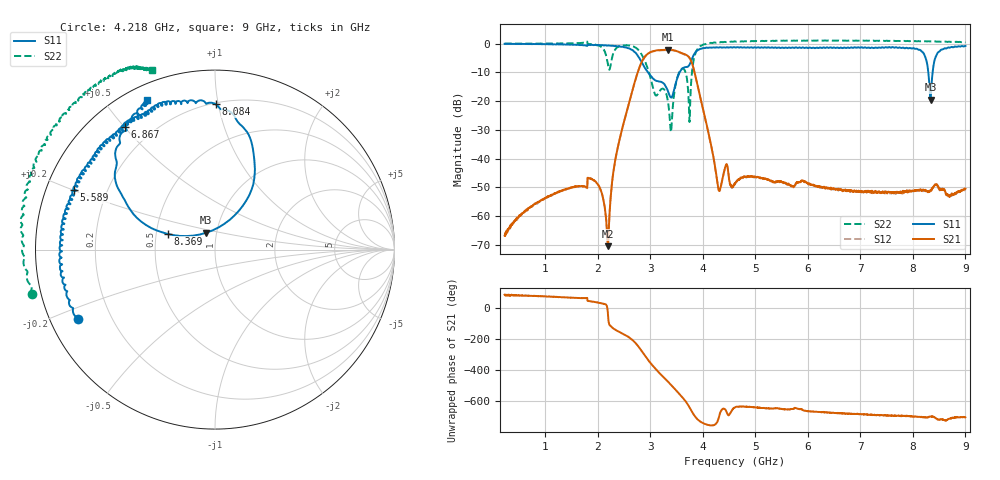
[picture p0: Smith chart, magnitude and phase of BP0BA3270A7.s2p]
!Agilent Technologies,E8358A,US41080443,A.07.50.56
!Agilent E8358A: A.07.50.56
!Date: Friday, July 21, 2017 20:19:28
!Correction: S11(Full 2 Port(1,2))
!S21(Full 2 Port(1,2))
!S12(Full 2 Port(1,2))
!S22(Full 2 Port(1,2))
!S2P File: Measurements: S11, S21, S12, S22:
# Hz S  dB  R 50
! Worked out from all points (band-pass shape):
!   1601 points, 225 MHz to 9 GHz, reference 50 ohm
!   highest |S21| = -2.10 dB at 3.329 GHz (marker M1); lowest = -70.5 dB at 2.194 GHz (marker M2)
!   |S21| within 3 dB of the highest: 2.874 GHz to 3.754 GHz (880.4 MHz wide, 26.6 % of centre)
!   lowest |S11| = -19.5 dB at 8.336 GHz (marker M3), VSWR 1.24, Z = 44.6 + j8.49 ohm
!   |S11| at or under -10 dB: 2.957 GHz to 3.557 GHz (600.2 MHz wide, 18.4 % of centre); 8.294 GHz to 8.376 GHz (81.74 MHz wide, 0.981 % of centre)
!   |S22| runs from -30.7 to 1.1 dB; largest |S21 - S12| = 0.013
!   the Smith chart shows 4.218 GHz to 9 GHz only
!   S11 on the Smith chart (normalised r, x): 4.218 GHz: 0.08, -0.24; 5.589 GHz: 0.08, +0.20; 6.867 GHz: 0.10, +0.50; 8.084 GHz: 0.21, +0.98; 8.369 GHz: 0.57, +0.11; 9 GHz: 0.06, +0.64
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2.25e8  -0.06 177.7  -66.77 84.5  -66.93 81.4  0.01 176.3
1.689328e9  -0.45 148.5  -49.57 63.0  -49.56 62.4  0.30 159.0
2.023875e9  -0.47 144.6  -49.59 32.3  -49.65 32.2  -0.69 91.9
2.193891e9  -0.64 135.6  -70.46 -48.2  -69.48 -43.5  -7.36 -8.7
2.347453e9  -0.80 122.5  -38.94 -144.4  -39.01 -144.2  -1.64 162.5
2.753297e9  -3.99 20.3  -10.29 119.6  -10.36 119.3  -1.83 73.8
2.906859e9  -8.73 -86.0  -4.28 47.1  -4.38 47.3  -6.50 32.0
3.153656e9  -13.08 -154.1  -2.26 -53.2  -2.37 -53.6  -17.19 -133.5
3.329156e9  -16.20 -159.7  -2.10 -113.4  -2.21 -114.0  -19.48 151.2
3.510141e9  -12.16 -97.5  -2.64 -178.7  -2.72 -179.3  -11.99 -116.2
3.691125e9  -8.13 -112.1  -3.97 108.6  -4.08 108.1  -11.52 -179.2
3.905016e9  -2.25 -121.9  -14.92 -0.4  -14.98 -1.0  -1.73 -118.0
4.217625e9  -1.33 -153.2  -41.25 -34.4  -41.26 -35.4  0.43 -166.3
4.6125e9  -1.30 -172.0  -48.64 78.5  -48.73 77.9  0.78 170.7
5.588719e9  -1.38 157.0  -48.56 65.2  -48.78 66.3  1.07 141.4
6.076828e9  -1.50 145.3  -49.06 51.9  -49.19 52.0  1.05 131.2
6.866578e9  -1.42 126.3  -51.57 36.2  -51.53 37.2  1.02 120.4
7.541156e9  -1.20 111.5  -51.50 25.5  -52.00 25.4  0.95 115.5
8.084109e9  -1.83 89.7  -50.94 18.7  -50.80 17.2  0.89 113.6
8.336391e9  -19.51 117.2  -50.97 19.5  -51.24 19.9  0.78 112.8
8.369297e9  -11.10 161.7  -50.17 21.0  -50.24 20.4  0.81 112.3
9e9  -0.76 114.3  -50.46 15.0  -50.57 16.7  0.53 109.3
